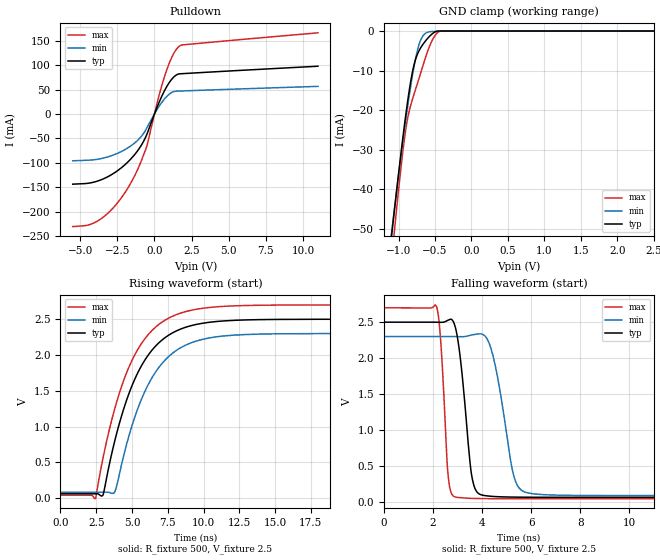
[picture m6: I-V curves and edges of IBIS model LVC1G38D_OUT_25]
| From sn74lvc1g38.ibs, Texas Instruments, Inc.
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[Model]   LVC1G38D_OUT_25
Model_type  Open_drain
Enable   Active-High
Vref =   2.5
Rref =   500
Cref =   30p
Vmeas =   1.25
| variable   typ   min   max
C_comp   3.98pF   3.13pF   5.06pF
| C_pulldown   7.90pF   4.71pF   12.60pF
| C_tri-state   3.98pF   3.13pF   5.06pF
[Temperature Range]   40   100   -40
| Ambient temperature   25   85   -40
[Voltage range]   2.5   2.3   2.7
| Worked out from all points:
|   slope of the pulldown table from 0 to 0.375 V, typ, clamps not added: 13.3 ohm
|   GND clamp passes 1 mA (typ) near -0.56 V on its own axis
|   rising waveform, R_fixture 500, V_fixture 2.5: 20-80 % time 2.68ns typ, 2.66ns min, 2.7ns max; typ from 0.061 V to 2.5 V
|   falling waveform, R_fixture 500, V_fixture 2.5: 20-80 % time 401ps typ, 626ps min, 244ps max; typ from 2.5 V to 0.061 V
[GND Clamp]
| LVC1G38D_OUT_25
|   Voltage   I(typ)   I(min)   I(max)
-5.5V     -916.4mA   -845.5mA   -1.045A
-1.12V    -55.82mA   -54.64mA   -62.42mA
-1.085V   -49.92mA   -49.21mA   -55.72mA
-1.055V   -44.94mA   -44.63mA   -50.09mA
-960mV    -29.8mA    -30.61mA   -33.36mA
-895mV    -20.34mA   -21.63mA   -24.12mA
-810mV    -10.37mA   -11.23mA   -17.25mA
-740mV    -5.781mA   -4.767mA   -13.16mA
-645mV    -2.839mA   -775.7uA   -7.523mA
-545mV    -806.1uA   -132uA     -2.586mA
-455mV    -12.65uA   -52.13uA   -238.9uA
2.5V      22.51pA    267pA      829.1pA
[Pulldown]
| LVC1G38D_OUT_25
|   Voltage   I(typ)   I(min)   I(max)
-5.5V     -143.8mA   -95.92mA   -230.8mA
-4.41V    -141.7mA   -94.67mA   -227.1mA
-3.55V    -134.4mA   -91.13mA   -213.8mA
-2.605V   -118.8mA   -82.16mA   -186.5mA
-1.71V    -95.98mA   -67.92mA   -147.7mA
-1.105V   -74.16mA   -53.22mA   -112.1mA
-550mV    -44.64mA   -30.61mA   -69.31mA
305mV     23.32mA    15.39mA    37.29mA
860mV     57.74mA    36.92mA    93.12mA
1.275V    74.94mA    45.66mA    122.7mA
1.665V    82.18mA    46.99mA    138.7mA
11V       97.87mA    56.59mA    166.3mA
[Ramp]
| LVC1G38D_OUT_25
| variable   typ   min   max
dV/dt_r   1.48/2.69E-09   1.34/2.66E-09   1.62/2.71E-09
dV/dt_f   1.49/4.15E-10   1.35/6.44E-10   1.62/2.50E-10
R_load = 500
[Rising Waveform]
| LVC1G38D_OUT_25
R_fixture =   500
C_fixture =   0
L_fixture =   0
V_fixture =   2.5
V_fixture_min = 2.3
V_fixture_max = 2.7
|   Time   V(typ)   V(min)   V(max)
0s        60.91mV    83.6mV     41.45mV
2.45ns    61.07mV    83.58mV    -5.822mV
2.98ns    47.94mV    83.68mV    565.5mV
3.75ns    762.9mV    72.95mV    1.218V
4.63ns    1.374V     758mV      1.756V
5.575ns   1.818V     1.34V      2.134V
6.5ns     2.092V     1.716V     2.362V
7.55ns    2.276V     1.977V     2.514V
11.54ns   2.478V     2.268V     2.681V
24.99ns   2.5V       2.3V       2.7V
[Falling Waveform]
| LVC1G38D_OUT_25
R_fixture =   500
C_fixture =   0
L_fixture =   0
V_fixture =   2.5
V_fixture_min = 2.3
V_fixture_max = 2.7
|   Time   V(typ)   V(min)   V(max)
0s        2.5V       2.3V       2.7V
2.15ns    2.5V       2.3V       2.71V
2.61ns    2.527V     2.3V       382.4mV
2.875ns   2.467V     2.299V     67.51mV
3.57ns    376.1mV    2.321V     45.91mV
3.975ns   94.18mV    2.337V     43.03mV
4.5ns     71.91mV    1.953V     41.89mV
5.3ns     63.56mV    349.7mV    41.51mV
5.79ns    62.1mV     128.5mV    41.47mV
24.99ns   60.91mV    83.6mV     41.45mV
